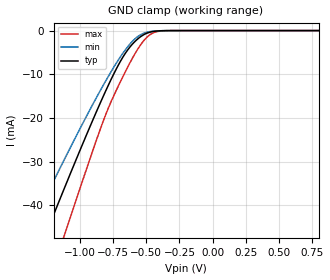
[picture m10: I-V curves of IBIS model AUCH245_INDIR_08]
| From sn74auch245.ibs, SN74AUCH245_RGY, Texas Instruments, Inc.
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[Model]   AUCH245_INDIR_08
Model_type  Input
Vinl=0.7
Vinh=0.8
| variable   typ   min   max
C_comp   2.64pF   2.25pF   2.97pF
[Temperature Range]   40   100   -40
| Ambient temperature   25   85   -40
[Voltage range]   0.8   0.8   0.8
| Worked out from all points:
|   GND clamp passes 1 mA (typ) near -0.52 V on its own axis
[GND Clamp]
| AUCH245_INDIR_08
|   Voltage   I(typ)   I(min)   I(max)
-3.6V     -229.3mA   -192.6mA   -273mA
-1.39V    -56.59mA   -46.25mA   -71.74mA
-1.245V   -45.56mA   -37.21mA   -58.43mA
-1.11V    -35.45mA   -28.97mA   -46.07mA
-835mV    -15.73mA   -13.06mA   -21.55mA
-710mV    -7.848mA   -6.681mA   -12.62mA
-595mV    -2.79mA    -2.165mA   -5.809mA
-535mV    -1.239mA   -831.9uA   -2.928mA
-480mV    -438.7uA   -276.8uA   -1.123mA
-430mV    -133.4uA   -89.21uA   -324.3uA
-350mV    -14.06uA   -12.12uA   -22.33uA
800mV     155pA      591pA      19.39pA
